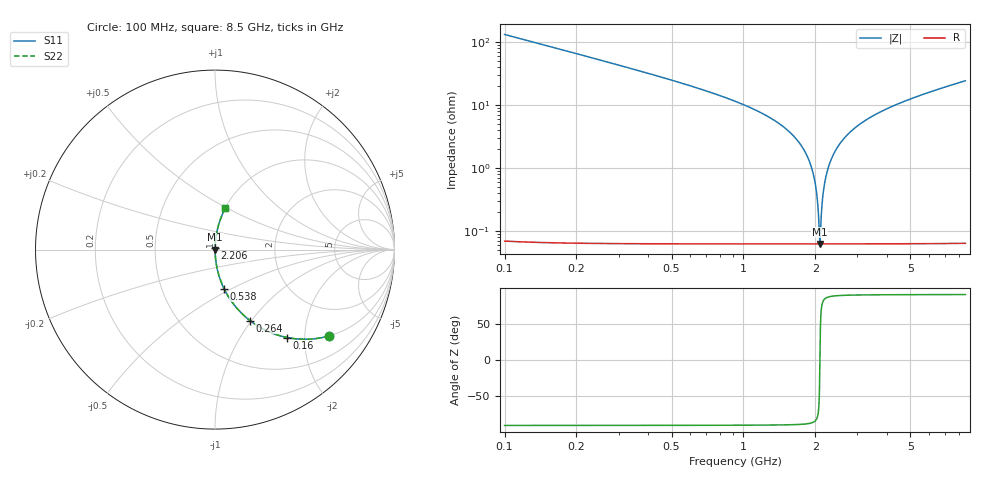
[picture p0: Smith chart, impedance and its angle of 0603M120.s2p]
! Created Wed Apr 18 16:37:41 2012
# hz S ma R 50
! 2 Port Network Data from SP1.SP block
! freq  magS11  angS11  magS21  angS21  magS12  angS12  magS22  angS22
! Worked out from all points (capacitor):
!   8401 points, 100 MHz to 8.5 GHz, reference 50 ohm
!   read as one part in series: C = 12.1 pF near 142 MHz
!   lowest |Z| = 63.1 mohm at 2.09 GHz (marker M1)
!   series resonance near 2.09 GHz, so ESL is about 480 pH
!   S11 on the Smith chart (normalised r, x): 100 MHz: 1.00, -2.63; 160 MHz: 1.00, -1.64; 264 MHz: 1.00, -0.98; 538 MHz: 1.00, -0.46; 2.206 GHz: 1.00, +0.01; 8.5 GHz: 1.00, +0.49
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1e8  0.7962 -37.2  0.6047 52.8  0.6047 52.8  0.7962 -37.2
1.6e8  0.6338 -50.6  0.773 39.3  0.773 39.3  0.6338 -50.6
2.64e8  0.4412 -63.7  0.8968 26.2  0.8968 26.2  0.4412 -63.7
5.38e8  0.2231 -76.9  0.9742 12.9  0.9742 12.9  0.2231 -76.9
1.5e9  0.04263 -86.7  0.9985 2.4  0.9985 2.4  0.04263 -86.7
1.745e9  0.02292 -87.1  0.9991 1.3  0.9991 1.3  0.02292 -87.1
1.908e9  0.01156 -86.2  0.9993 0.7  0.9993 0.7  0.01156 -86.2
1.998e9  0.005743 -83.4  0.9994 0.3  0.9994 0.3  0.005743 -83.4
2.028e9  0.003877 -80.4  0.9994 0.2  0.9994 0.2  0.003877 -80.4
2.064e9  0.001723 -68.4  0.9994 0.1  0.9994 0.1  0.001723 -68.4
2.09e9  0.0006309 -2.1  0.9994 0.0  0.9994 0.0  0.0006309 -2.1
2.115e9  0.001607 66.8  0.9994 -0.1  0.9994 -0.1  0.001607 66.8
2.16e9  0.004185 81.1  0.9994 -0.2  0.9994 -0.2  0.004185 81.1
2.206e9  0.006829 84.3  0.9993 -0.4  0.9993 -0.4  0.006829 84.3
2.302e9  0.01221 86.3  0.9993 -0.7  0.9993 -0.7  0.01221 86.3
2.444e9  0.01982 87.0  0.9992 -1.1  0.9992 -1.1  0.01982 87.0
2.9e9  0.04206 86.7  0.9985 -2.4  0.9985 -2.4  0.04206 86.7
3.479e9  0.06705 85.6  0.9971 -3.8  0.9971 -3.8  0.06705 85.6
4.3e9  0.09886 84.0  0.9945 -5.7  0.9945 -5.7  0.09886 84.0
5.7e9  0.1479 81.3  0.9884 -8.5  0.9884 -8.5  0.1479 81.3
7.1e9  0.1933 78.7  0.9805 -11.1  0.9805 -11.1  0.1933 78.7
8.5e9  0.2365 76.2  0.971 -13.7  0.971 -13.7  0.2365 76.2
